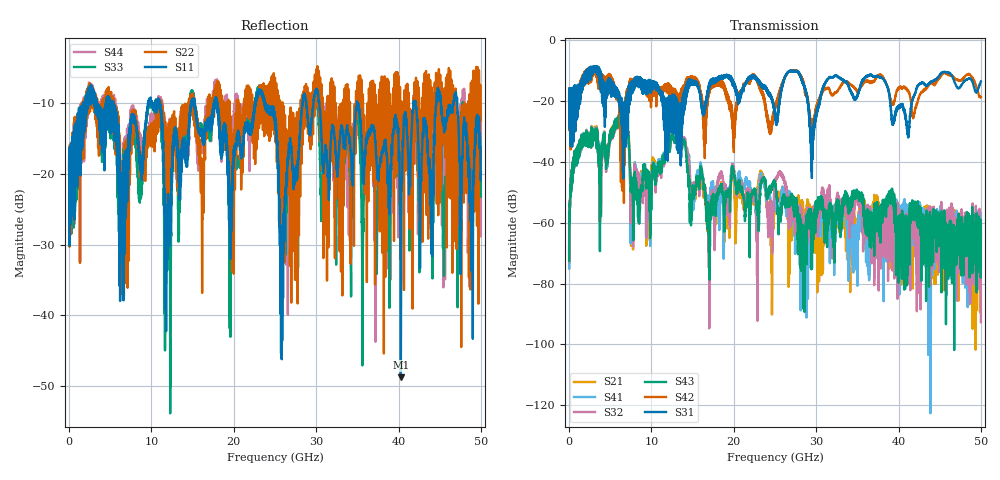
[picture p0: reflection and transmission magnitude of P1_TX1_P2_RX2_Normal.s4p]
!Keysight Technologies,N5225B,MY57041031,A.13.20.10
!Date: Friday, May 31, 2019 11:29:53
!Correction: S11(Full 4 Port(1,2,3,4))
!S12(Full 4 Port(1,2,3,4))
!S13(Full 4 Port(1,2,3,4))
!S14(Full 4 Port(1,2,3,4))
!S21(Full 4 Port(1,2,3,4))
!S22(Full 4 Port(1,2,3,4))
!S23(Full 4 Port(1,2,3,4))
!S24(Full 4 Port(1,2,3,4))
!S31(Full 4 Port(1,2,3,4))
!S32(Full 4 Port(1,2,3,4))
!S33(Full 4 Port(1,2,3,4))
!S34(Full 4 Port(1,2,3,4))
!S41(Full 4 Port(1,2,3,4))
!S42(Full 4 Port(1,2,3,4))
!S43(Full 4 Port(1,2,3,4))
!S44(Full 4 Port(1,2,3,4))
!S4P File: Measurements: <S11,S12,S13,S14>,
!<S21,S22,S23,S24>,
!<S31,S32,S33,S34>,
!<S41,S42,S43,S44>:
# Hz S  dB  R 50.0
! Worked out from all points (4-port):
!   5000 points, 10 MHz to 50 GHz, reference 50 ohm
!   strongest paths, dB at 10 MHz, 12.51 GHz, 25.01 GHz, 37.51 GHz, 50 GHz:
!     S31: -19.5, -29.2, -24.6, -11.8, -13.5
!     S42: -19.5, -16.0, -21.9, -11.5, -18.6
!     S43: -72.6, -31.0, -47.0, -60.4, -59.1
!     S32: -68.0, -30.8, -48.2, -72.0, -92.7
!     S41: -68.2, -30.3, -52.3, -59.7, -63.5
!     S21: -60.6, -30.6, -54.4, -53.8, -73.3
!   lowest |S11| = -48.8 dB at 40.28 GHz (marker M1), VSWR 1.01, Z = 50.4 + j0.00634 ohm
!   |S11| at or under -10 dB: 18.01 GHz to 22.61 GHz (4.595 GHz wide, 22.6 % of centre); 30.38 GHz to 34.94 GHz (4.562 GHz wide, 14 % of centre); 34.98 GHz to 41.81 GHz (6.836 GHz wide, 17.8 % of centre)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
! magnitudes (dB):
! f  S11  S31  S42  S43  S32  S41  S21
! 10 MHz  -20.0  -19.5  -19.5  -72.6  -68.0  -68.2  -60.6
! 6.24 GHz  -23.2  -23.5  -27.6  -23.3  -23.2  -23.1  -22.5
! 7.67 GHz  -11.7  -14.1  -13.1  -48.4  -51.0  -51.7  -56.6
! 13.2 GHz  -15.8  -36.2  -18.1  -29.5  -29.5  -29.6  -30.3
! 16.89 GHz  -12.8  -16.3  -18.7  -55.2  -58.3  -54.4  -60.3
! 40.28 GHz  -48.8  -21.8  -15.1  -63.7  -62.2  -59.2  -58.2
! 50 GHz  -19.8  -13.5  -18.6  -59.1  -92.7  -63.5  -73.3
